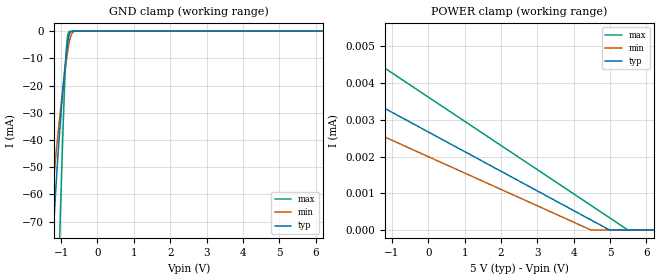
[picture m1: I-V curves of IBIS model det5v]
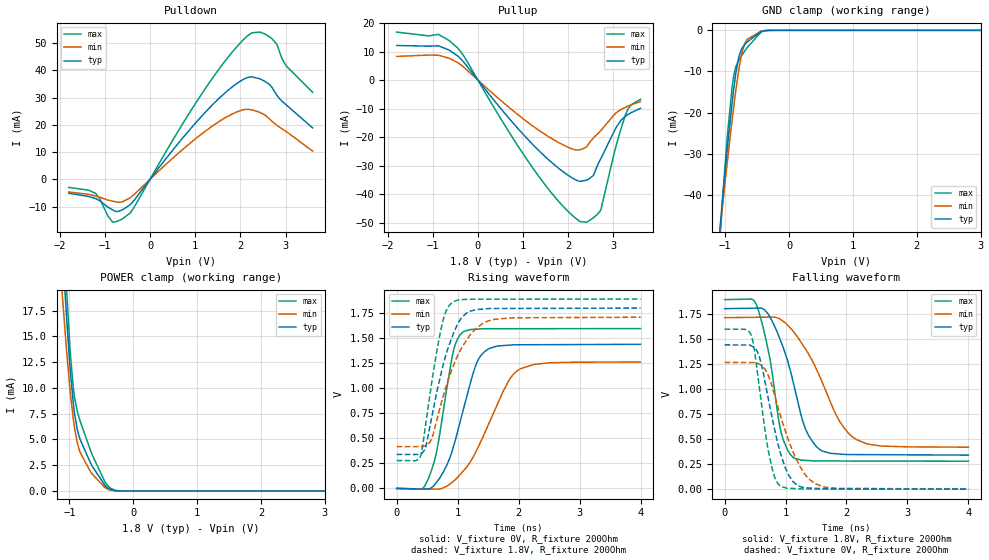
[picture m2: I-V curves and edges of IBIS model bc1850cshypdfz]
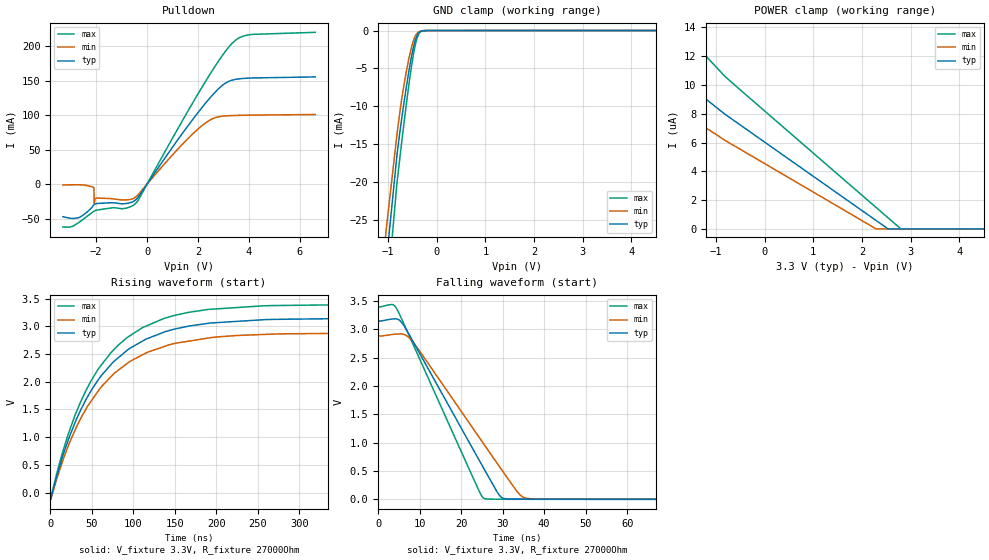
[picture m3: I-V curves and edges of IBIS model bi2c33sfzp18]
|Texas Instruments Incorporated
| Marketing part#   Package-type   #pins
| DS90UH929-Q1   QFN   64
[IBIS Ver]   4.1
[File name]   ds90uh929q1.ibs
[File Rev]   1.0
[Date]   10/06/2014
[Source]
| Texas Instruments Incorporated.
| 12500 TI Blvd
| Dallas, TX -75243
[Notes]   Revision History:
| Rev 1.0: 10/06/2014
| - Initial version of the model
| - Model generated from simulations in TISPICE
| - C_comp although listed in numerical order of value are
|   obtained from varying PVT conditions. For PVT conditions for
|   each specific value refer the buffer description under
|   respective [Model]. IBIS model user is responsible for using
|   appropriate C_comp to simulate for Signal Integrity.
| - Warnings regarding combined Non-monotonicity of various models have been
|   reviewd and considered minor and can be ignored.
[Disclaimer]
| This model is designed as an aid for customers of Texas Instruments.
| TI and its licensors and suppliers make no warranties, either expressed
| or implied, with respect to this  model, including the warranties of
| merchantability or fitness for a particular purpose. The model is
| provided solely on an "as is" basis. The entire risk as to its quality
| and performance is with the customer.
[Copyright]
 (C) Copyright 2014 Texas Instruments Incorporated.All rights reserved.
|   Device
[Component]   DS90UH929Q1
[Manufacturer]   TI
[Package]  |QFN   64
|   typ   min   max
R_pkg   0.067   0.027   0.083
L_pkg   0.937nH   0.593nH   1.143nH
C_pkg   0.144pF   0.126pF   0.200pF
[Pin]  signal_name   model_name   R_pin   L_pin   C_pin
1   CEC   bi2c33sfzp18   NA   NA   NA
2   RES0   NC   NA   NA   NA
3   VDDIO   POWER   NA   NA   NA
4   SDIN/GPIO0   bc1850cshypdfz   NA   NA   NA
5   SWC/GPIO1   bc1850cshypdfz   NA   NA   NA
6   SCLK/I2CSEL   bc1850cshypdfz   NA   NA   NA
7   VDDL11   POWER   NA   NA   NA
8   NC0   NC   NA   NA   NA
9   VDDA11   POWER   NA   NA   NA
10   NC1   NC   NA   NA   NA
11   NC2   NC   NA   NA   NA
12   NC3   NC   NA   NA   NA
13   INTB   bi2c33sfzp18   NA   NA   NA
14   SDA   bi2c33sfzp18   NA   NA   NA
15   SCL   bi2c33sfzp18   NA   NA   NA
16   MCLK   bc1850cshypdfz   NA   NA   NA
17   VDDP11   POWER   NA   NA   NA
18   MODE_SEL0   NC   NA   NA   NA
19   IDX   NC   NA   NA   NA
20   LFT   NC   NA   NA   NA
21   VDDHS11   POWER   NA   NA   NA
22   NC4   NC   NA   NA   NA
23   NC5   NC   NA   NA   NA
24   VDD18   POWER   NA   NA   NA
25   VDDS11   POWER   NA   NA   NA
26   DOUT-   hdcp_driver   NA   NA   NA
27   DOUT+   hdcp_driver   NA   NA   NA
28   VDDHS11   POWER   NA   NA   NA
29   RES1   NC   NA   NA   NA
30   RES2   NC   NA   NA   NA
31   PDB   IEC_ic18shypdfz   NA   NA   NA
32   MODE_SEL1   NC   NA   NA   NA
33   I2S_WC/GPIO7_REG   bc1850cshypdfz   NA   NA   NA
34   I2S_CLK/GPIO8_REG   bc1850cshypdfz   NA   NA   NA
35   I2S_DA/GPIO6_REG   bc1850cshypdfz   NA   NA   NA
36   I2S_DB/GPIO5_REG   bc1850cshypdfz   NA   NA   NA
37   I2S_DC/GPIO2   bc1850cshypdfz   NA   NA   NA
38   I2S_DD/GPIO3   bc1850cshypdfz   NA   NA   NA
39   X1   bc1850cshypdfz   NA   NA   NA
40   RES3   NC   NA   NA   NA
41   VDDL11   POWER   NA   NA   NA
42   HPD   bi2c5sfzp18   NA   NA   NA
43   RX_5V   det5v   NA   NA   NA
44   DDC_SDA   bi2c5sfzp18   NA   NA   NA
45   DDC_SCL   bi2c5sfzp18   NA   NA   NA
46   VDDIO   POWER   NA   NA   NA
47   NC6   NC   NA   NA   NA
48   NC7   NC   NA   NA   NA
49   IN_CLK-   lvdsin   NA   NA   NA
50   IN_CLK+   lvdsin   NA   NA   NA
51   VDD18   POWER   NA   NA   NA
52   VDDHA11   POWER   NA   NA   NA
53   RES4   NC   NA   NA   NA
54   VDDHA11   POWER   NA   NA   NA
55   IN_D0-   lvdsin   NA   NA   NA
56   IN_D0+   lvdsin   NA   NA   NA
57   VTERM   NC   NA   NA   NA
58   VDDHA11   POWER   NA   NA   NA
59   IN_D1-   lvdsin   NA   NA   NA
60   IN_D1+   lvdsin   NA   NA   NA
61   VDDHA11   POWER   NA   NA   NA
62   IN_D2-   lvdsin   NA   NA   NA
63   IN_D2+   lvdsin   NA   NA   NA
64   VDD18   POWER   NA   NA   NA
[Diff Pin]  inv_pin  vdiff  tdelay_typ tdelay_min tdelay_max
50   49   200mV   NA   NA   NA
56   55   200mV   NA   NA   NA
60   59   200mV   NA   NA   NA
63   62   200mV   NA   NA   NA
27   26   NA   NA   NA   NA
23   22   NA   NA   NA   NA
| Models and submodels in the file (7): det5v (Input), bc1850cshypdfz (I/O), bi2c33sfzp18 (I/O_open_drain), bi2c5sfzp18 (I/O_open_drain), hdcp_driver (Output), lvdsin (Input), IEC_ic18shypdfz (Input)
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|   Model
[Model]   det5v
Model_type   Input
Vinl = 1.5
Vinh = 3.5
|   typ   min   max
C_comp   0.213pF   0.192pF   0.234pF
[Voltage Range]   5   4.5   5.5
[Temperature Range]   27   105   -40
[Power Clamp Reference]   5   4.5   5.5
[GND Clamp Reference]   0   0   0
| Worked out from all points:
|   GND clamp passes 1 mA (typ) near -0.77 V on its own axis
|   POWER clamp passes 1 mA (typ) near -4.25 V on its own axis
[GND Clamp]
|   Voltage   I(typ)   I(min)   I(max)
-5V       -1.183A    -1A        -2.22A
-1.31V    -98.67mA   -73.95mA   -209.5mA
-1.25V    -83.13mA   -62.66mA   -178.7mA
-1.19V    -68.35mA   -52.56mA   -148.3mA
-1.04V    -36.85mA   -31.81mA   -76.24mA
-1.025V   -34.16mA   -29.95mA   -69.45mA
-920mV    -17.03mA   -17.6mA    -25.77mA
-875mV    -10.65mA   -12.77mA   -11.24mA
-830mV    -5.307mA   -8.405mA   -2.714mA
-755mV    -618.4uA   -2.83mA    -88.57uA
-620mV    -2.926uA   -44.04uA   -544.5nA
10V       0A         0A         0A
[POWER Clamp]
|   Voltage   I(typ)   I(min)   I(max)
-5V       106.1mA    280.9mA    8.174uA
-4.025V   5.714uA    96.68mA    7.01uA
-3.845V   5.306uA    68.8mA     6.823uA
-3.2V     4.733uA    81.99uA    6.164uA
-1.25V    3.342uA    2.558uA    4.446uA
4.465V    277.9nA    2.966nA    676.4nA
4.975V    4.186nA    0A         340.1nA
5.515V    0A         0A         0A
10V       0A         0A         0A
|   Model
[Model]   bc1850cshypdfz
Model_type   I/O
Polarity   Non-Inverting
Enable   Active-Low
Vinl = 0.54
Vinh = 1.26
Vmeas = 0.9
Vref = 0
Cref = 1pF
Rref = 100000
|   typ   min   max
C_comp   0.255pF   0.213pF   0.269pF
[Voltage Range]   1.8   1.71   1.89
[Temperature Range]   27   105   -40
[Pullup Reference]   1.8   1.71   1.89
[Pulldown Reference]   0   0   0
[Power Clamp Reference]   1.8   1.71   1.89
[GND Clamp Reference]   0   0   0
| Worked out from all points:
|   slope of the pulldown table from 0 to 0.27 V, typ, clamps not added: 46.3 ohm
|   slope of the pullup table from 0 to 0.27 V, typ, clamps not added: 50 ohm
|   GND clamp passes 1 mA (typ) near -0.50 V on its own axis
|   POWER clamp passes 1 mA (typ) near -0.49 V on its own axis
|   falling waveform, V_fixture 1.8V, R_fixture 200Ohm: 20-80 % time 407ps typ, 619ps min, 266ps max; typ from 1.8 V to 0.34 V
|   rising waveform, V_fixture 0V, R_fixture 200Ohm: 20-80 % time 394ps typ, 588ps min, 261ps max; typ from 0 V to 1.44 V
|   rising waveform, V_fixture 1.8V, R_fixture 200Ohm: 20-80 % time 358ps typ, 459ps min, 253ps max; typ from 0.34 V to 1.8 V
|   falling waveform, V_fixture 0V, R_fixture 200Ohm: 20-80 % time 317ps typ, 428ps min, 226ps max; typ from 1.44 V to 0 V
[Pulldown]
|   Voltage   I(typ)   I(min)   I(max)
-1.8V     -5.11mA    -4.631mA   -2.961mA
-1.206V   -7.051mA   -6.135mA   -5.191mA
-828mV    -11.22mA   -8.014mA   -15.69mA
-698.4mV  -11.73mA   -8.432mA   -15.19mA
-444.6mV  -9.401mA   -6.834mA   -12.42mA
1.262V    25.27mA    18.14mA    34.22mA
1.888V    34.75mA    24.49mA    48mA
2.261V    37.58mA    25.49mA    53.77mA
2.698V    33.8mA     21.3mA     51.63mA
2.806V    30.88mA    19.85mA    49.61mA
3.017V    27.32mA    17.52mA    41.58mA
3.6V      18.87mA    10.39mA    31.92mA
[GND Clamp]
|   Voltage   I(typ)   I(min)   I(max)
-1.8V     -223.9mA   -200.7mA   -257.6mA
-1.076V   -47.33mA   -48.12mA   -49.68mA
-1.044V   -41.55mA   -43.28mA   -42.02mA
-963mV    -28.24mA   -31.62mA   -25.27mA
-892.8mV  -17.9mA    -22.11mA   -14.13mA
-860.4mV  -13.67mA   -17.98mA   -10.65mA
-833.4mV  -10.55mA   -14.73mA   -8.857mA
-784.8mV  -6.37mA    -9.464mA   -7.168mA
-736.2mV  -4.37mA    -5.373mA   -5.995mA
-693mV    -3.477mA   -3.168mA   -5.026mA
-444.6mV  -340uA     -254.2uA   -548.7uA
3.6V      0A         0A         0A
[Pullup]
|   Voltage   I(typ)   I(min)   I(max)
-1.8V     12.14mA    8.304mA    16.83mA
-882mV    12mA       8.707mA    16.02mA
-444.6mV  8.432mA    6.129mA    11.22mA
1.224V    -22.74mA   -16.21mA   -31.03mA
1.791V    -30.98mA   -21.94mA   -42.61mA
2.266V    -35.51mA   -24.44mA   -49.63mA
2.552V    -33.5mA    -20.35mA   -48.35mA
2.714V    -27.73mA   -17.84mA   -45.69mA
3.033V    -17.46mA   -11.9mA    -24.61mA
3.265V    -12.67mA   -9.532mA   -12.25mA
3.389V    -11.44mA   -8.711mA   -8.682mA
3.6V      -9.885mA   -7.498mA   -6.719mA
[POWER Clamp]
|   Voltage   I(typ)   I(min)   I(max)
-1.8V     109.9mA    89.55mA    132.5mA
-1.109V   23.6mA     19mA       28mA
-1.098V   22.44mA    18.08mA    26.57mA
-1.044V   16.93mA    13.72mA    19.76mA
-984.6mV  11.68mA    9.57mA     13.45mA
-936mV    8.429mA    6.912mA    9.947mA
-871.2mV  5.886mA    4.608mA    7.656mA
-828mV    4.956mA    3.707mA    6.743mA
-666mV    2.688mA    1.855mA    3.893mA
-417.6mV  406.7uA    236.2uA    668.5uA
-207mV    3.345uA    2.309uA    8.785uA
3.6V      0A         0A         0A
[Ramp]
R_load = 200
|   typ   min   max
dV/dt_r   0.863003/3.93107e-10   0.757132/5.8424e-10   0.957265/2.6067e-10
dV/dt_f   0.876119/4.04883e-10   0.774779/6.16626e-10   0.966532/2.64126e-10
[Falling Waveform]
V_fixture = 1.8V
V_fixture_min = 1.71V
V_fixture_max = 1.89V
R_fixture = 200Ohm
C_fixture = 0F
|   Time   V(typ)   V(min)   V(max)
0s        1.8V       1.71V      1.89V
518.4ps   1.805V     1.714V     1.845V
734.2ps   1.727V     1.716V     1.332V
930.6ps   1.463V     1.687V     557.7mV
1.132ns   1.05V      1.569V     314.6mV
1.321ns   610.8mV    1.404V     287.3mV
1.512ns   420.8mV    1.189V     281.4mV
1.834ns   352.8mV    735.4mV    281.1mV
2.098ns   345.1mV    520.9mV    280.9mV
4ns       339.8mV    418.7mV    279.1mV
[Rising Waveform]
V_fixture = 0V
V_fixture_min = 0V
V_fixture_max = 0V
R_fixture = 200Ohm
C_fixture = 0F
|   Time   V(typ)   V(min)   V(max)
0s        43.88uV    45.6uV     39.57uV
407.4ps   -5.274mV   -4.097mV   -5.943mV
514.4ps   -6.67mV    -5.185mV   88.97mV
674.4ps   77.6mV     -6.812mV   425.6mV
931.8ps   417.4mV    71.71mV    1.374V
1.087ns   773mV      170.6mV    1.561V
1.379ns   1.325V     465.6mV    1.592V
1.826ns   1.429V     1.063V     1.594V
2.031ns   1.434V     1.195V     1.594V
4ns       1.438V     1.262V     1.595V
[Rising Waveform]
V_fixture = 1.8V
V_fixture_min = 1.71V
V_fixture_max = 1.89V
R_fixture = 200Ohm
C_fixture = 0F
|   Time   V(typ)   V(min)   V(max)
0s        339.5mV    417.2mV    279mV
392.2ps   347.3mV    417.8mV    321.7mV
478.3ps   418.8mV    428.7mV    647.6mV
573.1ps   702.9mV    493.9mV    1.047V
725.3ps   1.137V     837.6mV    1.582V
811.2ps   1.339V     1.017V     1.771V
921.3ps   1.529V     1.21V      1.861V
1.153ns   1.752V     1.485V     1.887V
1.514ns   1.795V     1.674V     1.889V
4ns       1.8V       1.709V     1.89V
[Falling Waveform]
|Gnd
V_fixture = 0V
V_fixture_min = 0V
V_fixture_max = 0V
R_fixture = 200Ohm
C_fixture = 0F
|   Time   V(typ)   V(min)   V(max)
0s        1.439V     1.264V     1.596V
441.3ps   1.428V     1.262V     1.528V
573.7ps   1.317V     1.246V     1V
719ps     898.1mV    1.13V      381.5mV
818ps     603.1mV    944.2mV    127.2mV
919.3ps   353.3mV    728.9mV    29.24mV
1.119ns   77.52mV    379mV      6.793mV
1.317ns   14.51mV    148.3mV    2.243mV
1.507ns   8.165mV    49.04mV    2.095mV
4ns       247.5uV    1.121mV    153.4uV
|   Model
[Model]   bi2c33sfzp18
Model_type   I/O_open_drain
Polarity   Non-Inverting
Enable   Active-Low
Vinl = 0.99
Vinh = 2.31
Vmeas = 1.65
Vref = 3.3
Cref = 1pF
Rref = 27000
|   typ   min   max
C_comp   0.176pF   0.126pF   0.258pF
[Voltage Range]   3.3   3   3.6
[Temperature Range]   27   105   -40
[Pullup Reference]   3.3   3   3.6
[Pulldown Reference]   -0   0   0
[Power Clamp Reference]   3.3   3   3.6
[GND Clamp Reference]   0   0   0
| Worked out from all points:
|   slope of the pulldown table from 0 to 0.495 V, typ, clamps not added: 18.4 ohm
|   GND clamp passes 1 mA (typ) near -0.42 V on its own axis
|   falling waveform, V_fixture 3.3V, R_fixture 27000Ohm: 20-80 % time 14.4ns typ, 16.3ns min, 12.5ns max; typ from 3.15 V to 0.002 V
|   rising waveform, V_fixture 3.3V, R_fixture 27000Ohm: 20-80 % time 74.2ns typ, 75.3ns min, 72.3ns max; typ from 0.002 V to 3.15 V
[Pulldown]
|   Voltage   I(typ)   I(min)   I(max)
-3.3V     -47.2mA    -1.083mA   -62.22mA
-2.676V   -48.56mA   -863.5uA   -55.57mA
-2.102V   -30.79mA   -4.436mA   -39.66mA
-2.082V   -29.95mA   -5.797mA   -39.23mA
-2.072V   -29.62mA   -27.7mA    -39.03mA
-1.983V   -28.19mA   -20.23mA   -37.75mA
-409.2mV  -21.6mA    -17.57mA   -26.53mA
2.095V    108.5mA    83.11mA    137mA
2.927V    142.6mA    98.57mA    185.4mA
3.482V    152.3mA    99.81mA    209.3mA
4.135V    154.2mA    100.3mA    217.5mA
6.6V      155.8mA    101.2mA    220.5mA
[GND Clamp]
|   Voltage   I(typ)   I(min)   I(max)
-3.3V     -395.1mA   -358.4mA   -431.4mA
-1.073V   -34.01mA   -28.65mA   -41.1mA
-1.023V   -29.88mA   -25.55mA   -35.34mA
-815.1mV  -16.47mA   -13.76mA   -20.15mA
-755.7mV  -13.43mA   -10.78mA   -16.84mA
-666.6mV  -9.369mA   -7.031mA   -12.03mA
-557.7mV  -4.897mA   -3.353mA   -6.586mA
-478.5mV  -2.265mA   -1.382mA   -3.226mA
-409.2mV  -767.1uA   -424.1uA   -1.152mA
-349.8mV  -203.3uA   -115.4uA   -303.3uA
-171.6mV  -3.042uA   -2.771uA   -3.369uA
6.6V      0A         0A         0A
[POWER Clamp]
|   Voltage   I(typ)   I(min)   I(max)
-3.3V     21.2uA     14.63uA    63.88uA
-3.142V   19.24uA    13.73uA    51.16uA
-2.449V   14.07uA    10.88uA    23.45uA
-2.34V    13.51uA    10.5uA     21.45uA
-1.845V   11.31uA    8.857uA    15.7uA
-1.498V   9.955uA    7.778uA    13.35uA
-1.34V    9.385uA    7.323uA    12.49uA
-815.1mV  7.974uA    6.16uA     10.6uA
2.284V    602.6nA    14.88nA    1.511uA
2.531V    13.85nA    0A         786nA
2.798V    0A         0A         3.367nA
6.6V      0A         0A         0A
[Ramp]
R_load = 27000
|   typ   min   max
dV/dt_r   1.88543/7.3565e-08   1.7266/7.46981e-08   2.03482/7.21349e-08
dV/dt_f   1.88614/1.43789e-08   1.72733/1.63195e-08   2.0354/1.25056e-08
[Falling Waveform]
V_fixture = 3.3V
V_fixture_min = 3V
V_fixture_max = 3.6V
R_fixture = 27000Ohm
C_fixture = 0F
|   Time   V(typ)   V(min)   V(max)
0s        3.146V     2.881V     3.394V
3.669ns   3.182V     2.91V      3.428V
5.997ns   3.085V     2.912V     3.126V
8.895ns   2.718V     2.726V     2.654V
24.35ns   690.1mV    1.093V     144.6mV
26.24ns   443.5mV    892.6mV    7.46mV
29.87ns   27.89mV    510.9mV    3.486mV
34.22ns   5.385mV    77.27mV    2.766mV
37.38ns   3.442mV    9.621mV    2.634mV
700ns     2.262mV    2.554mV    1.998mV
[Rising Waveform]
V_fixture = 3.3V
V_fixture_min = 3V
V_fixture_max = 3.6V
R_fixture = 27000Ohm
C_fixture = 0F
|   Time   V(typ)   V(min)   V(max)
0s        2.262mV    2.554mV    1.998mV
328.7ps   -17.03mV   659.2uV    -32.39mV
619.8ps   -110.6mV   -121.7mV   -103.4mV
14.42ns   629.9mV    548mV      707.2mV
29.47ns   1.249V     1.114V     1.381V
57ns      2.017V     1.817V     2.21V
91.32ns   2.55V      2.315V     2.781V
136.4ns   2.891V     2.631V     3.138V
256.6ns   3.119V     2.853V     3.369V
700ns     3.145V     2.88V      3.393V
